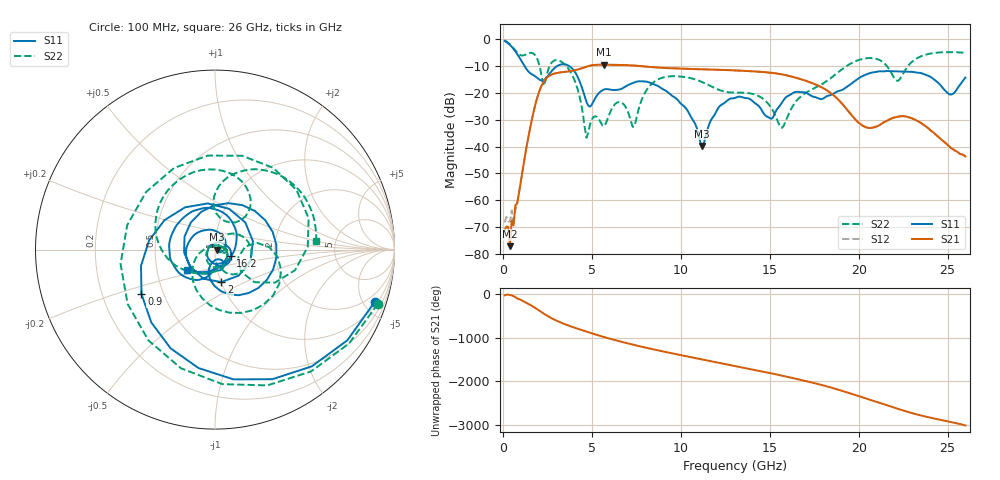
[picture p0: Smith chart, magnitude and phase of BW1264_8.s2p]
!Keysight Technologies,N5245B,MY57181159,A.13.60.06
!Date: Friday, December 18, 2020 23:52:18
!Correction: S11(Full 2 Port(1,2))
!S21(Full 2 Port(1,2))
!S12(Full 2 Port(1,2))
!S22(Full 2 Port(1,2))
!S2P File: Measurements: S11, S21, S12, S22:
# Hz S  dB  R 50
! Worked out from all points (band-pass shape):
!   260 points, 100 MHz to 26 GHz, reference 50 ohm
!   highest |S21| = -9.42 dB at 5.7 GHz (marker M1); lowest = -77.1 dB at 400 MHz (marker M2)
!   |S21| within 3 dB of the highest: 3.121 GHz to 15.03 GHz (11.91 GHz wide, 131 % of centre)
!   lowest |S11| = -39.7 dB at 11.2 GHz (marker M3), VSWR 1.02, Z = 51 - j0.0523 ohm
!   |S11| at or under -10 dB: 1.224 GHz to 3.045 GHz (1.821 GHz wide, 85.3 % of centre); 3.74 GHz to end of sweep
!   |S22| runs from -36.7 to -0.4 dB; largest |S21 - S12| = 0.0005
!   S11 on the Smith chart (normalised r, x): 100 MHz: 1.27, -6.04; 900 MHz: 0.38, -0.24; 2 GHz: 1.00, -0.38; 16.2 GHz: 1.19, -0.08; 26 GHz: 0.71, -0.17
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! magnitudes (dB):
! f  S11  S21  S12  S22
! 100 MHz  -0.6  -71.2  -68.3  -0.4
! 400 MHz  -2.0  -77.1  -68.0  -1.8
! 900 MHz  -6.4  -57.7  -57.3  -5.5
! 2 GHz  -14.7  -20.3  -20.3  -8.4
! 2.3 GHz  -15.2  -15.7  -15.7  -17.3
! 3.6 GHz  -9.5  -12.0  -12.0  -10.2
! 4.5 GHz  -19.1  -10.6  -10.6  -27.7
! 4.7 GHz  -23.2  -10.2  -10.2  -36.7
! 5.7 GHz  -18.7  -9.4  -9.4  -32.3
! 6.6 GHz  -18.6  -9.5  -9.5  -23.4
! 7.4 GHz  -16.0  -9.8  -9.8  -32.4
! 8.8 GHz  -17.7  -10.5  -10.5  -14.7
! 11.2 GHz  -39.7  -11.2  -11.2  -15.9
! 13.1 GHz  -21.7  -11.6  -11.6  -19.8
! 15.1 GHz  -29.6  -12.5  -12.5  -25.6
! 15.7 GHz  -23.5  -13.1  -13.1  -33.0
! 16.2 GHz  -20.5  -13.8  -13.8  -26.0
! 17.4 GHz  -21.2  -16.3  -16.3  -18.6
! 20.4 GHz  -13.1  -32.8  -32.8  -7.1
! 21.7 GHz  -11.8  -29.9  -29.9  -11.0
! 25.2 GHz  -20.6  -40.6  -40.6  -4.7
! 26 GHz  -14.2  -43.7  -43.6  -5.0
